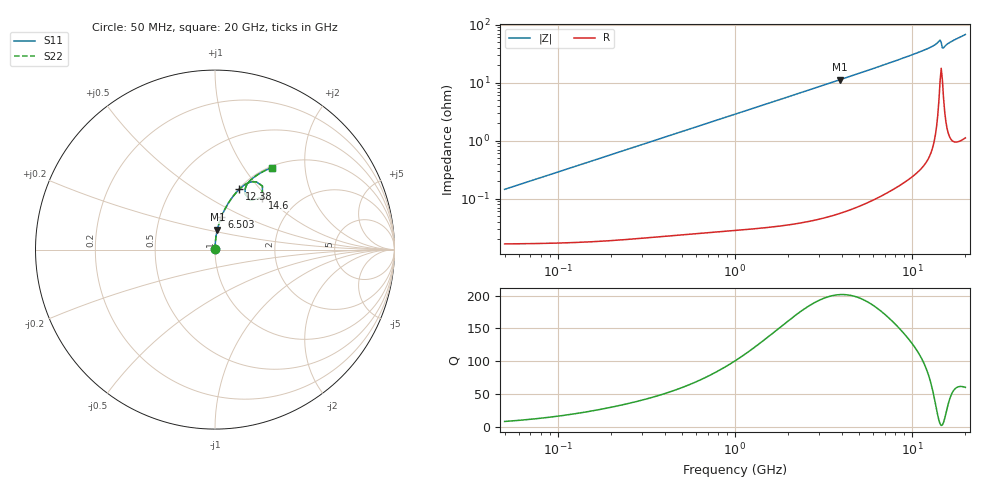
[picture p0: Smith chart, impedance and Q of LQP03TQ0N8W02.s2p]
!Murata Part Number: LQP03TQ0N8W02
!These Parameters are Measured in Series Mode Connection
!  o--[Z]--o
!Port1  Port2
!  o-------o
!Freq. Start=50[MHz] Stop=20[GHz], 401[Steps]
# Hz S RI R 50
!Freq.(Hz) S11(Real) S11(Imag) S21(Real) S21(Imag) S12(Real) S12(Imag) S22(Real) S22(Imag)
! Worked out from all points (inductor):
!   401 points, 50 MHz to 20 GHz, reference 50 ohm
!   read as one part in series: L = 457 pH near 51.52 MHz
!   highest Q = 202 at 3.908 GHz (marker M1), where L = 456 pH
!   S11 on the Smith chart (normalised r, x): 50 MHz: 1.00, +0.00; 6.503 GHz: 1.00, +0.38; 12.38 GHz: 1.01, +0.78; 14.6 GHz: 1.35, +0.92; 20 GHz: 1.02, +1.35
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5e7  0.000168 0.00144  0.9998 -0.00144  0.9998 -0.00144  0.000168 0.00144
1.364002e8  0.000192 0.00391  0.9998 -0.00391  0.9998 -0.00391  0.000192 0.00391
3.721004e8  0.000333 0.0106  0.9997 -0.0106  0.9997 -0.0106  0.000333 0.0106
1e9  0.00109 0.0284  0.9989 -0.0284  0.9989 -0.0284  0.00109 0.0284
1.714689e9  0.0027 0.0487  0.9973 -0.0487  0.9973 -0.0487  0.0027 0.0487
2.728004e9  0.00642 0.0773  0.9936 -0.0773  0.9936 -0.0773  0.00642 0.0773
3.908127e9  0.0129 0.1104  0.9871 -0.1104  0.9871 -0.1104  0.0129 0.1104
6.503449e9  0.0354 0.1821  0.9646 -0.1821  0.9646 -0.1821  0.0354 0.1821
7.442007e9  0.0465 0.2075  0.9535 -0.2075  0.9535 -0.2075  0.0465 0.2075
1.004137e10  0.0857 0.2761  0.9143 -0.2761  0.9143 -0.2761  0.0857 0.2761
1.238412e10  0.136 0.3365  0.864 -0.3365  0.864 -0.3365  0.136 0.3365
1.334722e10  0.1679 0.3627  0.8321 -0.3627  0.8321 -0.3627  0.1679 0.3627
1.396067e10  0.2064 0.378  0.7936 -0.378  0.7936 -0.378  0.2064 0.378
1.417136e10  0.231 0.3768  0.769 -0.3768  0.769 -0.3768  0.231 0.3768
1.460232e10  0.2634 0.2891  0.7366 -0.2891  0.7366 -0.2891  0.2634 0.2891
1.504638e10  0.1681 0.3101  0.8319 -0.3101  0.8319 -0.3101  0.1681 0.3101
1.527346e10  0.1676 0.3372  0.8324 -0.3372  0.8324 -0.3372  0.1676 0.3372
1.550395e10  0.1738 0.355  0.8262 -0.355  0.8262 -0.355  0.1738 0.355
1.597544e10  0.1894 0.3776  0.8106 -0.3776  0.8106 -0.3776  0.1894 0.3776
1.670968e10  0.213 0.3996  0.787 -0.3996  0.787 -0.3996  0.213 0.3996
1.855685e10  0.2702 0.436  0.7298 -0.436  0.7298 -0.436  0.2702 0.436
2e10  0.3159 0.4567  0.6841 -0.4567  0.6841 -0.4567  0.3159 0.4567
